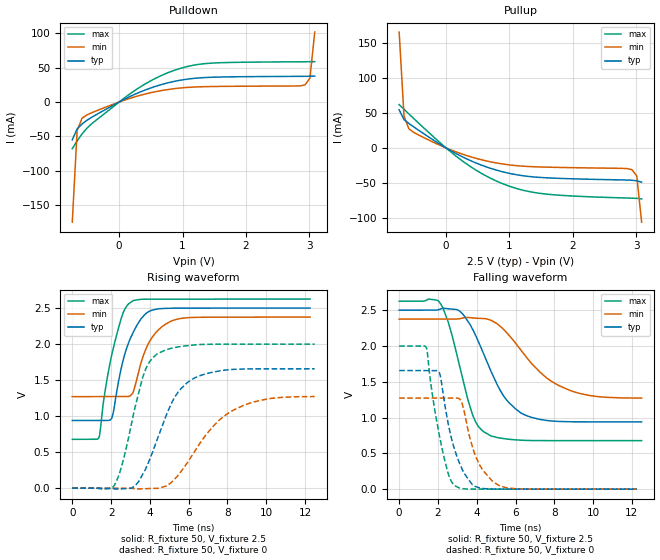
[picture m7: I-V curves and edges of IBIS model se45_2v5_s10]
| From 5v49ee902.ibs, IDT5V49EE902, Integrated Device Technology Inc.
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[Model]   se45_2v5_s10
Model_type   Output
Polarity   Non-Inverting
|   typ   min   max
C_comp   2pF   1.5pF   2.5pF
Vmeas = 1.25V
Rref = 50
Cref = 0
Vref = 1.25V
|   typ   min   max
[Voltage range]   2.5V   2.375V   2.625V
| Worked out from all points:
|   slope of the pulldown table from 0 to 0.375 V, typ, clamps not added: 23.2 ohm
|   slope of the pullup table from 0 to 0.375 V, typ, clamps not added: 21 ohm
|   rising waveform, R_fixture 50, V_fixture 2.5: 20-80 % time 951ps typ, 985ps min, 850ps max; typ from 0.939 V to 2.5 V
|   falling waveform, R_fixture 50, V_fixture 2.5: 20-80 % time 1.65ns typ, 2.29ns min, 1.11ns max; typ from 2.5 V to 0.939 V
|   rising waveform, R_fixture 50, V_fixture 0: 20-80 % time 1.55ns typ, 2.24ns min, 1.07ns max; typ from 0 V to 1.66 V
|   falling waveform, R_fixture 50, V_fixture 0: 20-80 % time 891ps typ, 940ps min, 781ps max; typ from 1.66 V to 0 V
[Pulldown]
|Voltage   I (typ)   I (min)   I (max)
|Note, modeling breaks down at 250mA and above.  This is well beyond the functional   |
|operating range of the device.  Should this scenario occur, catastrophic failure and   |
|possible damage to the device and/or board is of higher concern than the I-V curve   |
|behavior.  The IBIS checker will flag currents in excess of 10A with warnings.  Lines   |
|with currents in excess of 0.35 A have been commented out.  The points still remain|
|available to the user if the user desires to use them.   |
|-2.50000e+00   -4.54709e+01   -3.63694e+01   -6.07959e+01
|-2.42347e+00   -4.32502e+01   -3.46594e+01   -5.77053e+01
|-2.34694e+00   -4.10314e+01   -3.29511e+01   -5.46170e+01
|-2.27041e+00   -3.88148e+01   -3.12446e+01   -5.15313e+01
|-2.19388e+00   -3.66007e+01   -2.95401e+01   -4.84486e+01
|-2.11735e+00   -3.43893e+01   -2.78380e+01   -4.53691e+01
|-2.04082e+00   -3.21809e+01   -2.61384e+01   -4.22934e+01
|-1.96429e+00   -2.99761e+01   -2.44418e+01   -3.92219e+01
|-1.88776e+00   -2.77753e+01   -2.27484e+01   -3.61555e+01
|-1.81122e+00   -2.55791e+01   -2.10589e+01   -3.30948e+01
|-1.73469e+00   -2.33884e+01   -1.93737e+01   -3.00411e+01
|-1.65816e+00   -2.12042e+01   -1.76937e+01   -2.69958e+01
|-1.58163e+00   -1.90279e+01   -1.60198e+01   -2.39607e+01
|-1.50510e+00   -1.68611e+01   -1.43533e+01   -2.09385e+01
|-1.42857e+00   -1.47065e+01   -1.26960e+01   -1.79331e+01
|-1.35204e+00   -1.25675e+01   -1.10500e+01   -1.49501e+01
|-1.27551e+00   -1.04495e+01   -9.41889e+00   -1.19989e+01
|-1.19898e+00   -8.36102e+00   -7.80755e+00   -9.09553e+00
|-1.12245e+00   -6.31683e+00   -6.22400e+00   -6.27207e+00
|-1.04592e+00   -4.34540e+00   -4.68188e+00   -3.60463e+00
|-9.69388e-01   -2.51112e+00   -3.20700e+00   -1.33260e+00
|-8.92857e-01   -9.89892e-01   -1.85502e+00   -2.01598e-01
|-8.16327e-01   -1.92135e-01   -7.61074e-01   -8.24374e-02
-739.8mV  -54.82mA   -174.4mA   -67.73mA
-663.3mV  -39mA      -41.68mA   -56.5mA
-586.7mV  -31.96mA   -23.62mA   -46.47mA
-433.7mV  -22.15mA   -15.6mA    -31.55mA
255.1mV   11.54mA    7.746mA    17.23mA
637.8mV   24.55mA    16.14mA    37.26mA
943.9mV   31.29mA    20.16mA    48.22mA
1.173V    34.28mA    21.72mA    53.44mA
1.48V     36mA       22.52mA    56.56mA
2.934V    37.31mA    24.91mA    58.47mA
3.01V     37.39mA    34.58mA    58.51mA
3.087V    37.69mA    101.5mA    58.57mA
| 3.16327e+00   3.94370e-02   3.90716e-01   5.87161e-02
| 3.23980e+00   5.34569e-02   9.26332e-01   5.92247e-02
| 3.31633e+00   1.87777e-01   1.58664e+00   6.05142e-02
| 3.39286e+00   7.03900e-01   2.30650e+00   6.31621e-02
| 3.46939e+00   1.49296e+00   3.05902e+00   8.17834e-02
| 3.54592e+00   2.39302e+00   3.83167e+00   3.62573e-01
| 3.62245e+00   3.34512e+00   4.61786e+00   1.23067e+00
| 3.69898e+00   4.32630e+00   5.41369e+00   2.35283e+00
| 3.77551e+00   5.32579e+00   6.21672e+00   3.56536e+00
| 3.85204e+00   6.33779e+00   7.02533e+00   4.82080e+00
| 3.92857e+00   7.35883e+00   7.83838e+00   6.10084e+00
| 4.00510e+00   8.38670e+00   8.65504e+00   7.39669e+00
| 4.08163e+00   9.41993e+00   9.47469e+00   8.70352e+00
| 4.15816e+00   1.04574e+01   1.02969e+01   1.00184e+01
| 4.23469e+00   1.14984e+01   1.11212e+01   1.13394e+01
| 4.31122e+00   1.25424e+01   1.19474e+01   1.26653e+01
| 4.38776e+00   1.35888e+01   1.27751e+01   1.39952e+01
| 4.46429e+00   1.46373e+01   1.36044e+01   1.53282e+01
| 4.54082e+00   1.56877e+01   1.44348e+01   1.66640e+01
| 4.61735e+00   1.67397e+01   1.52665e+01   1.80021e+01
| 4.69388e+00   1.77932e+01   1.60991e+01   1.93422e+01
| 4.77041e+00   1.88479e+01   1.69326e+01   2.06841e+01
| 4.84694e+00   1.99037e+01   1.77670e+01   2.20275e+01
| 4.92347e+00   2.09606e+01   1.86021e+01   2.33723e+01
| 5.00000e+00   2.20184e+01   1.94379e+01   2.47183e+01
[Pullup]
|Voltage   I (typ)   I (min)   I (max)
|Note, modeling breaks down at 250mA and above.  This is well beyond the functional   |
|operating range of the device.  Should this scenario occur, catastrophic failure and   |
|possible damage to the device and/or board is of higher concern than the I-V curve   |
|behavior.  The IBIS checker will flag currents in excess of 10A with warnings.  Lines   |
|with currents in excess of 0.35 A have been commented out.  The points still remain|
|available to the user if the user desires to use them.   |
|-2.50000e+00   2.19765e+01   1.80472e+01   2.68517e+01
|-2.42347e+00   2.09191e+01   1.72127e+01   2.55048e+01
|-2.34694e+00   1.98626e+01   1.63791e+01   2.41589e+01
|-2.27041e+00   1.88071e+01   1.55463e+01   2.28141e+01
|-2.19388e+00   1.77528e+01   1.47145e+01   2.14705e+01
|-2.11735e+00   1.66997e+01   1.38838e+01   2.01283e+01
|-2.04082e+00   1.56480e+01   1.30543e+01   1.87877e+01
|-1.96429e+00   1.45980e+01   1.22261e+01   1.74489e+01
|-1.88776e+00   1.35497e+01   1.13995e+01   1.61122e+01
|-1.81122e+00   1.25036e+01   1.05747e+01   1.47780e+01
|-1.73469e+00   1.14600e+01   9.75186e+00   1.34466e+01
|-1.65816e+00   1.04193e+01   8.93142e+00   1.21187e+01
|-1.58163e+00   9.38215e+00   8.11380e+00   1.07950e+01
|-1.50510e+00   8.34928e+00   7.29955e+00   9.47668e+00
|-1.42857e+00   7.32178e+00   6.48942e+00   8.16516e+00
|-1.35204e+00   6.30119e+00   5.68442e+00   6.86272e+00
|-1.27551e+00   5.28973e+00   4.88602e+00   5.57292e+00
|-1.19898e+00   4.29091e+00   4.09630e+00   4.30185e+00
|-1.12245e+00   3.31066e+00   3.31857e+00   3.06117e+00
|-1.04592e+00   2.36002e+00   2.55827e+00   1.87712e+00
|-9.69388e-01   1.46263e+00   1.82537e+00   8.26238e-01
|-8.92857e-01   6.79721e-01   1.14025e+00   1.77022e-01
|-8.16327e-01   1.78304e-01   5.50947e-01   7.20287e-02
-739.8mV  54.64mA    166.3mA    62.19mA
-663.3mV  40.61mA    45.96mA    55.4mA
-586.7mV  35.13mA    27.42mA    48.78mA
-204.1mV  11.53mA    8.292mA    16.47mA
255.1mV   -12.67mA   -8.857mA   -18.54mA
561.2mV   -24.84mA   -17.08mA   -36.7mA
943.9mV   -35.45mA   -23.78mA   -53.18mA
1.25V     -40.42mA   -26.48mA   -61.53mA
1.556V    -42.81mA   -27.59mA   -66.09mA
2.934V    -46.44mA   -31.28mA   -72.19mA
3.01V     -47.21mA   -40.39mA   -72.48mA
3.087V    -49.28mA   -106.7mA   -73.28mA
| 3.16327e+00   -5.35776e-02   -4.94236e-01   -7.58575e-02
| 3.23980e+00   -6.85824e-02   -1.43626e+00   -8.09811e-02
| 3.31633e+00   -2.12479e-01   -2.71822e+00   -8.81300e-02
| 3.39286e+00   -1.02359e+00   -4.15794e+00   -9.69442e-02
| 3.46939e+00   -2.55073e+00   -5.67974e+00   -1.18777e-01
| 3.54592e+00   -4.38708e+00   -7.25021e+00   -4.69271e-01
| 3.62245e+00   -6.35927e+00   -8.85247e+00   -2.14689e+00
| 3.69898e+00   -8.40369e+00   -1.04769e+01   -4.62063e+00
| 3.77551e+00   -1.04921e+01   -1.21177e+01   -7.36117e+00
| 3.85204e+00   -1.26099e+01   -1.37710e+01   -1.02197e+01
| 3.92857e+00   -1.47486e+01   -1.54342e+01   -1.31429e+01
| 4.00510e+00   -1.69029e+01   -1.71053e+01   -1.61066e+01
| 4.08163e+00   -1.90692e+01   -1.87829e+01   -1.90980e+01
| 4.15816e+00   -2.12452e+01   -2.04660e+01   -2.21093e+01
| 4.23469e+00   -2.34289e+01   -2.21537e+01   -2.51357e+01
| 4.31122e+00   -2.56192e+01   -2.38455e+01   -2.81738e+01
| 4.38776e+00   -2.78148e+01   -2.55407e+01   -3.12215e+01
| 4.46429e+00   -3.00151e+01   -2.72389e+01   -3.42769e+01
| 4.54082e+00   -3.22195e+01   -2.89399e+01   -3.73388e+01
| 4.61735e+00   -3.44273e+01   -3.06432e+01   -4.04061e+01
| 4.69388e+00   -3.66382e+01   -3.23486e+01   -4.34782e+01
| 4.77041e+00   -3.88519e+01   -3.40560e+01   -4.65543e+01
| 4.84694e+00   -4.10679e+01   -3.57652e+01   -4.96340e+01
| 4.92347e+00   -4.32862e+01   -3.74759e+01   -5.27168e+01
| 5.00000e+00   -4.55064e+01   -3.91880e+01   -5.58024e+01
[Ramp]
|   typ   min   max
dV/dt_r   0.936/0.951n   0.662/0.984n   1.168/0.849n
dV/dt_f   0.951/1.674n   0.675/2.319n   1.186/1.129n
R_load =   50
[Rising Waveform]
R_fixture = 50
V_fixture = 2.5   |Vcc_typ
V_fixture_min = 2.375 |Vcc_min
V_fixture_max = 2.625 |Vcc_max
C_fixture = 0.0p
| Time   typ   min   max
0s        939.3mV    1.271V     677.7mV
1.379ns   939.3mV    1.271V     705.4mV
1.634ns   939.3mV    1.271V     1.249V
1.957ns   946.9mV    1.271V     1.752V
2.176ns   1.14V      1.271V     2.01V
2.625ns   1.779V     1.271V     2.435V
3.161ns   2.174V     1.348V     2.606V
3.952ns   2.453V     2.02V      2.623V
5.113ns   2.498V     2.32V      2.624V
12.26ns   2.5V       2.375V     2.625V
[Falling Waveform]
R_fixture = 50
V_fixture = 2.5   |Vcc_typ
V_fixture_min = 2.375 |Vcc_min
V_fixture_max = 2.625 |Vcc_max
C_fixture = 0.0p
| Time   typ   min   max
0s        2.5V       2.375V     2.625V
2.148ns   2.517V     2.375V     2.585V
2.55ns    2.519V     2.375V     2.316V
3.067ns   2.497V     2.379V     1.774V
3.762ns   2.247V     2.392V     1.055V
4.473ns   1.815V     2.381V     784.1mV
5.456ns   1.274V     2.211V     703.9mV
6.596ns   1.024V     1.83V      680.4mV
8.861ns   941.2mV    1.374V     677.8mV
12.5ns    939.4mV    1.272V     677.7mV
[Rising Waveform]
R_fixture = 50
V_fixture = 0
C_fixture = 0.0p
| Time   typ   min   max
0s        96.64nV    102.5nV    85.59nV
2.167ns   -10.44mV   21.36nV    38.43mV
2.602ns   -8.119mV   19.28uV    359.1mV
3.633ns   191.6mV    -8.642mV   1.542V
4.377ns   675.7mV    -2.794mV   1.864V
5.329ns   1.283V     139mV      1.954V
6.371ns   1.538V     537mV      1.991V
7.5ns     1.624V     925.9mV    1.999V
8.762ns   1.654V     1.142V     1.999V
12.5ns    1.657V     1.272V     1.999V
[Falling Waveform]
R_fixture = 50
V_fixture = 0
C_fixture = 0.0p
| Time   typ   min   max
0s        1.657V     1.272V     1.999V
1.397ns   1.657V     1.272V     1.98V
2.081ns   1.625V     1.272V     739.7mV
2.521ns   925.1mV    1.272V     223.1mV
2.873ns   543.3mV    1.272V     47.01mV
3.216ns   297.3mV    1.225V     8.618mV
3.762ns   65.89mV    600.8mV    985.1uV
4.345ns   8.592mV    254.6mV    719.1uV
5.1ns     1.24mV     59.45mV    541.1uV
12.26ns   51.08uV    95.06uV    28.72uV
